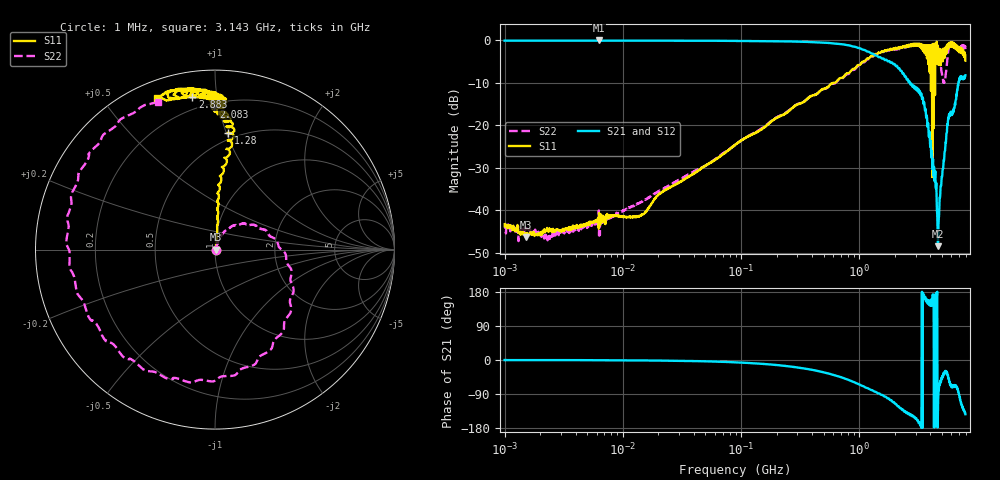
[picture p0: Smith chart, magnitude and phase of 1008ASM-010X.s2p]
!s-Parameter Generated by FASTRON Sdn. Bhd.
!FASTRON P/N : 1008ASM-010X
!Keysight Technologies: E5071C_MY46733604_B.14.02
!Date: Tue Nov 21 10:53:41 2023
!Version  :Rev00  Wed Nov 22 15:27:18 2023
!Data & Calibration Information:
!Freq  S11:SOLT2(ON)  S21:SOLT2(ON)  S12:SOLT2(ON)  S22:SOLT2(ON)
!PortZ  Port1:50+j0  Port2:50+j0
!When reading reference impedance value at option line is always used.
! Remarks : This data is being provided solely for informational purposes.
# Hz S dB R 50
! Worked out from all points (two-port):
!   1599 points, 1 MHz to 7.923 GHz, reference 50 ohm
!   highest |S21| = -0.01 dB at 6.301 MHz (marker M1); lowest = -48.5 dB at 4.633 GHz (marker M2)
!   |S21| within 3 dB of the highest: start of sweep to 1.255 GHz
!   lowest |S11| = -46.3 dB at 1.505 MHz (marker M3), VSWR 1.01, Z = 50.5 - j0.0273 ohm
!   |S11| at or under -10 dB: start of sweep to 614.1 MHz; 4.049408 GHz to 4.061026 GHz (11.62 MHz wide, 0.286 % of centre); 4.139 GHz to 4.176 GHz (36.51 MHz wide, 0.878 % of centre)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
!   |S22| runs from -47.3 to -0.6 dB; largest |S21 - S12| = 0.01
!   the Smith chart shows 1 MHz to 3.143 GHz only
!   S11 on the Smith chart (normalised r, x): 1 MHz: 1.01, -0.00; 1.28 GHz: 0.45, +1.02; 2.083 GHz: 0.22, +0.96; 2.883 GHz: 0.13, +0.85; 3.143 GHz: 0.07, +0.68
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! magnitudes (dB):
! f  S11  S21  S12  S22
! 1 MHz  -43.3  -0.1  -0.1  -43.8
! 1.505 MHz  -46.3  0.0  -0.1  -44.7
! 2.337 MHz  -44.8  -0.1  -0.1  -46.2
! 4.479 MHz  -43.5  -0.1  -0.1  -44.3
! 6.301 MHz  -40.7  0.0  0.0  -46.0
! 13.97 MHz  -41.3  -0.1  -0.1  -38.2
! 19.95 MHz  -36.3  -0.1  -0.1  -35.6
! 89.01 MHz  -24.6  -0.1  -0.1  -24.7
! 398.5 MHz  -13.0  -0.4  -0.4  -13.0
! 1.28 GHz  -3.7  -3.1  -3.1  -3.9
! 1.784 GHz  -2.3  -4.8  -4.9  -2.4
! 2.083 GHz  -2.0  -6.0  -6.0  -2.2
! 2.883 GHz  -1.3  -10.7  -10.7  -1.1
! 3.143 GHz  -0.9  -11.7  -11.7  -1.1
! 3.71 GHz  -1.2  -18.2  -18.2  -1.6
! 4.197 GHz  -3.4  -29.3  -29.3  -1.0
! 4.633 GHz  -1.3  -48.5  -48.6  -1.5
! 4.773 GHz  -5.3  -38.7  -38.7  -3.5
! 5.192 GHz  -4.2  -28.2  -28.2  -9.6
! 5.724 GHz  -0.7  -18.4  -18.4  -1.7
! 7.075 GHz  -1.8  -9.3  -9.3  -1.8
! 7.923 GHz  -4.8  -8.2  -8.2  -2.0
